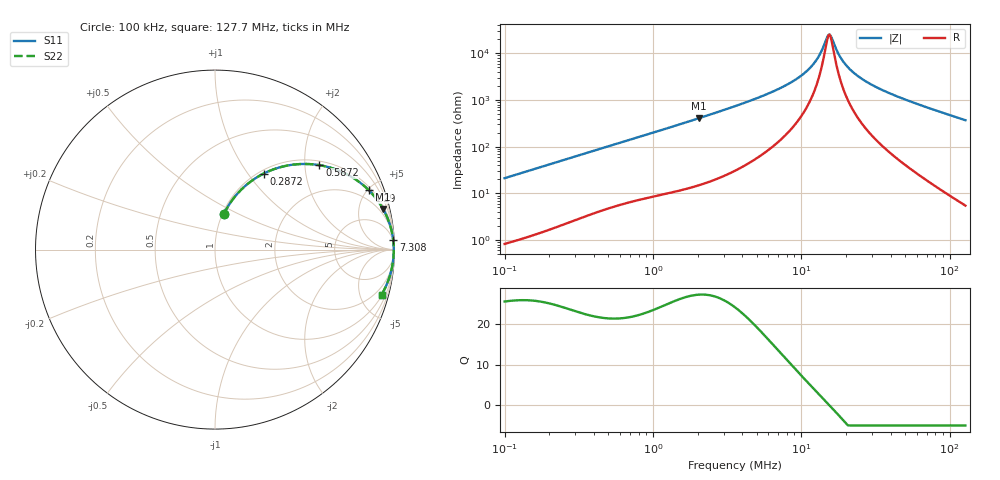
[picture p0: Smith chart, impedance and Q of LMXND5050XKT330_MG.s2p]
! LMXND5050XKT330_MG  S-PARAMETER MODEL  ( General Type )
! Model Generated by TAIYO YUDEN Corporation (http://www.ty-top.com)
! Version 1.0
! TAIYO YUDEN Control No. 191023NI43SB-FBB
! Copyright(c) 2019 TAIYO YUDEN CO.,LTD. All Rights Reserved.
! Product Description (link to TY-COMPAS)
! https://ds.yuden.co.jp/TYCOMPAS/or/detail?pn=LMXND5050XKT330MMG&u=M
! Products Name : Inductors
! Characteristics :
!  Inductance : 33 uH , SRF(min) : 10 MHz , DC Resistance(max) : 0.2925 Ohm
!  Rated Current : Saturation :1150 mA , Temp Rise : 800 mA
!  Case Size : 4.9 x 4.9 / 0.193 x 0.193 [mm/inch] , Thickness : 3 / 0.118 [mm/inch]
!  (Conditions: Temperature = 25 degC , DC Bias Current/Voltage = 0A / 0V)
! External Node Assignments :
!  1  o---GGG---o  2
! GND o---------o GND
! Frequency Range : 0.1MHz  -  127.746476MHz  [ 402 STEP ]
# MHz S RI R 50
! Freq[MHz].  S11 Real  S11 Imag  S21 Real  S21 Imag  S12 Real  S12 Imag  S22 Real  S22 Imag
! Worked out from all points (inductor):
!   401 points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, 100 kHz to 127.7 MHz, reference 50 ohm
!   read as one part in series: L = 33.5 uH near 103.6 kHz
!   highest Q = 27.3 at 2.053 MHz (marker M1), where L = 31.7 uH
!   self-resonance near 15.21 MHz
!   S11 on the Smith chart (normalised r, x): 100 kHz: 1.02, +0.42; 287.2 kHz: 1.05, +1.19; 587.2 kHz: 1.11, +2.38; 1.29 MHz: 1.20, +5.12; 7.308 MHz: 4, +37; 127.7 MHz: 1.11, -7.39
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0.1  0.05 0.1993  0.95 -0.1993  0.95 -0.1993  0.05 0.1993
0.174077  0.1268 0.3138  0.8732 -0.3138  0.8732 -0.3138  0.1268 0.3138
0.287201  0.2702 0.4232  0.7298 -0.4232  0.7298 -0.4232  0.2702 0.4232
0.33137  0.3259 0.4472  0.6741 -0.4472  0.6741 -0.4472  0.3259 0.4472
0.587248  0.5821 0.4704  0.4179 -0.4704  0.4179 -0.4704  0.5821 0.4704
1.098062  0.8171 0.3664  0.1829 -0.3664  0.1829 -0.3664  0.8171 0.3664
1.289792  0.8584 0.3294  0.1416 -0.3294  0.1416 -0.3294  0.8584 0.3294
2.053206  0.9364 0.2263  0.0636 -0.2263  0.0636 -0.2263  0.9364 0.2263
3.574164  0.9767 0.1316  0.0233 -0.1316  0.0233 -0.1316  0.9767 0.1316
7.308182  0.9928 0.0538  0.00717 -0.0538  0.00717 -0.0538  0.9928 0.0538
9.72889  0.9949 0.0315  0.00507 -0.0315  0.00507 -0.0315  0.9949 0.0315
11.84371  0.9957 0.0177  0.00431 -0.0177  0.00431 -0.0177  0.9957 0.0177
13.18509  0.9959 0.0105  0.00407 -0.0105  0.00407 -0.0105  0.9959 0.0105
14.94322  0.9961 0.00217  0.00394 -0.00217  0.00394 -0.00217  0.9961 0.00217
15.48731  0.9961 -0.000185  0.00392 0.000185  0.00392 0.000185  0.9961 -0.000185
16.05121  0.9961 -0.00254  0.00392 0.00254  0.00392 0.00254  0.9961 -0.00254
18.51973  0.996 -0.012  0.00404 0.012  0.00404 0.012  0.996 -0.012
21.75342  0.9956 -0.023  0.00441 0.023  0.00441 0.023  0.9956 -0.023
27.9415  0.9944 -0.0413  0.00558 0.0413  0.00558 0.0413  0.9944 -0.0413
39.24654  0.9911 -0.0704  0.00885 0.0704  0.00885 0.0704  0.9911 -0.0704
67.1085  0.978 -0.133  0.022 0.133  0.022 0.133  0.978 -0.133
127.7465  0.9286 -0.2502  0.0714 0.2502  0.0714 0.2502  0.9286 -0.2502
